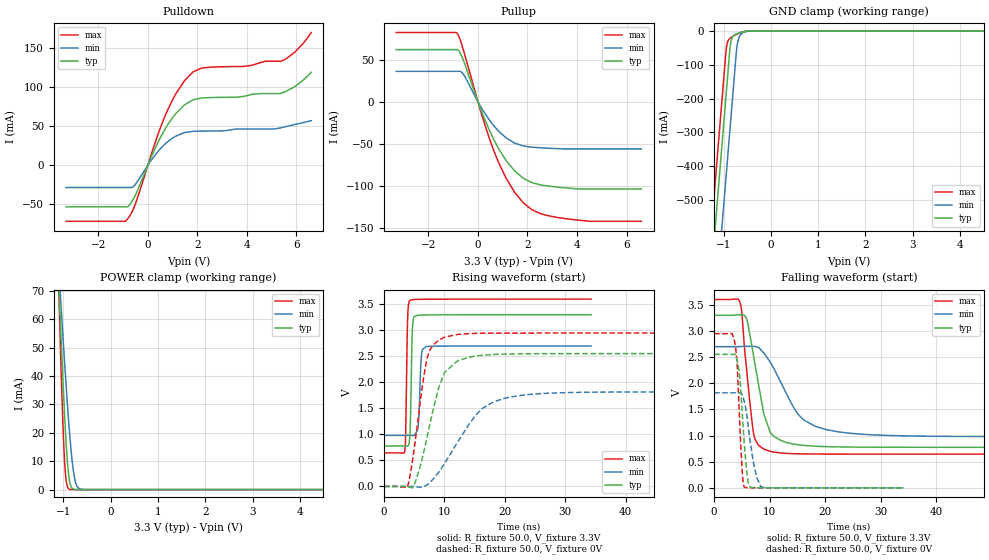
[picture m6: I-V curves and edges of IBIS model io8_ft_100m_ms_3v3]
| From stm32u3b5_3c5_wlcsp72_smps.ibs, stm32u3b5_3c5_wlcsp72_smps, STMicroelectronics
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[Model]   io8_ft_100m_ms_3v3
Model_type I/O
Polarity   Non-Inverting
Enable   Active-Low
| CAP_THRESHOLD on pad IOFT is "UDTCAPC" :
| Rising=30.0% of vddiom   Falling=70.0% of vddiom
| C_comp min and max val. don't necessarily correlate with the min and max pvt
| but are the smallest and greatest pad capacitance found.
| var   typ   min   max
C_comp   3.79549pF  3.74406pF  3.79817pF
|C_comp_pullup   2.32784pF  2.17308pF  2.40204pF
|C_comp_pulldown   1.46765pF  1.57099pF  1.39613pF
Vinl = 1.35V
Vinh = 1.8V
Vmeas = 1.65V   | Reference voltage for timing measurements
Cref  = 50.0pF   | Timing specification test load capacitance value
Rref  = 1.0MOhm   | Timing specification test load resistance value
Vref  = 1.815V   | Timing specification test load voltage
[Model Spec]
| TIME_THRESHOLD on pin ZIV11 is "CMOS" :
| Rising=50.0% of vdd   Falling=50.0% of vdd
Vinl 1.27950V 1.06950V 1.36550V
Vinh 1.78950V 1.51350V 1.89450V
| variable   typ   min   max
[Temperature Range] 25.0 130.0 -40.0
| variable   typ   min   max
[Voltage Range] 3.3V 2.7V 3.6V
| variable   typ   min   max
[POWER Clamp Reference] 3.3V 2.7V 3.6V
| variable   typ   min   max
[GND Clamp Reference] 0V 0V 0V
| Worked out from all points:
|   slope of the pulldown table from 0 to 0.495 V, typ, clamps not added: 14.3 ohm
|   slope of the pullup table from 0 to 0.495 V, typ, clamps not added: 13.8 ohm
|   GND clamp passes 1 mA (typ) near -0.50 V on its own axis
|   POWER clamp passes 1 mA (typ) near -0.83 V on its own axis
|   rising waveform, R_fixture 50.0, V_fixture 3.3V: 20-80 % time 257ps typ, 338ps min, 239ps max; typ from 0.776 V to 3.3 V
|   falling waveform, R_fixture 50.0, V_fixture 3.3V: 20-80 % time 2.72ns typ, 5.55ns min, 1.62ns max; typ from 3.3 V to 0.776 V
|   rising waveform, R_fixture 50.0, V_fixture 0V: 20-80 % time 3.27ns typ, 6.29ns min, 2.11ns max; typ from 0 V to 2.55 V
|   falling waveform, R_fixture 50.0, V_fixture 0V: 20-80 % time 1.01ns typ, 1.53ns min, 771ps max; typ from 2.55 V to 0 V
[POWER Clamp]
-3.3V     1.126A     769.5mA    1.647A
-1.1V     75.38mA    79.63mA    73.18mA
-1.09V    71.2mA     76.8mA     67.14mA
-1.08V    67.05mA    73.98mA    61.2mA
-1.06V    58.89mA    68.38mA    49.67mA
-1.01V    39.47mA    54.71mA    24.03mA
-970mV    25.49mA    44.18mA    9.257mA
-930mV    13.81mA    34.16mA    2.168mA
-870mV    3.251mA    20.56mA    140.6uA
-760mV    67.19uA    3.98mA     739.8nA
-630mV    518.7nA    149.1uA    1.803nA
6.6V      0A         0A         0A
[GND Clamp]
-3.3V     -4.191A    -4.432A    -4.059A
-1.25V    -706mA     -946.8mA   -573.6mA
-950mV    -196mA     -436.8mA   -63.63mA
-940mV    -179mA     -419.8mA   -50.26mA
-910mV    -128mA     -368.8mA   -31.05mA
-850mV    -37.37mA   -266.8mA   -20.53mA
-810mV    -18.79mA   -198.8mA   -16.88mA
-720mV    -8.735mA   -51.28mA   -10.12mA
-680mV    -6.635mA   -22.61mA   -7.598mA
-630mV    -4.51mA    -9.474mA   -4.925mA
-400mV    -114.4uA   -369.6uA   -46.93uA
6.6V      2.22nA     299.7nA    1.002nA
| variable   typ   min   max
[Pullup Reference] 3.3V 2.7V 3.6V
| variable   typ   min   max
[Pulldown Reference] 0V 0V 0V
[Pullup]
-3.3V     61.97mA    36.11mA    82.22mA
-840mV    61.97mA    36.11mA    81.38mA
-720mV    58.1mA     36.07mA    73.72mA
-570mV    48mA       31.88mA    59.76mA
170mV     -13.41mA   -8.675mA   -17.26mA
800mV     -53.86mA   -33.82mA   -69.73mA
1.14V     -69.93mA   -42.96mA   -90.97mA
1.48V     -82.17mA   -49.14mA   -107.6mA
2.17V     -96.08mA   -54mA      -128.2mA
2.85V     -100.3mA   -55.28mA   -135.6mA
3.88V     -103.2mA   -56.04mA   -140.2mA
6.6V      -103.8mA   -56.04mA   -142.1mA
[Pulldown]
-3.3V     -53.27mA   -28.52mA   -71.84mA
-840mV    -53.27mA   -28.52mA   -69.65mA
-500mV    -38.18mA   -24.47mA   -49.51mA
460mV     32.61mA    19.53mA    43.99mA
800mV     51.7mA     30.09mA    70.55mA
1.14V     66.56mA    37.47mA    92mA
1.48V     77.24mA    41.82mA    108.3mA
1.83V     83.91mA    43.43mA    119.6mA
2.17V     86.16mA    43.73mA    124.5mA
5.39V     92.36mA    48.12mA    133.3mA
5.93V     100.6mA    52.1mA     144.5mA
6.6V      119.1mA    57.05mA    170mA
[Ramp]
dV/dt_r 1.53142V/3.19498ns 1.09015V/6.22627ns 1.76896V/2.11107ns
dV/dt_f 1.51461V/2.56951ns 1.03188V/5.48087ns 1.77292V/1.61927ns
R_load = 50.0
| Removed startup time: 0s 0s 0s  .
| Removed end time: 34.25ns.
[Rising Waveform]
R_fixture   = 50.0
V_fixture   = 3.3V
V_fixture_min = 2.7V
V_fixture_max = 3.6V
0s        775.7mV    980.2mV    645.1mV
3.45ns    775.7mV    980.2mV    693.9mV
3.9ns     773.7mV    980.2mV    3.174V
4.3ns     998.1mV    980.2mV    3.573V
4.65ns    2.858V     979.9mV    3.587V
5ns       3.263V     977.5mV    3.593V
5.7ns     3.29V      1.21V      3.595V
6.25ns    3.294V     2.568V     3.597V
7ns       3.296V     2.691V     3.597V
34.25ns   3.3V       2.7V       3.6V
| Removed startup time: 0s 0s 0s  .
| Removed end time: 99.25ns.
[Falling Waveform]
R_fixture   = 50.0
V_fixture   = 3.3V
V_fixture_min = 2.7V
V_fixture_max = 3.6V
0s        3.3V       2.7V       3.6V
4.65ns    3.308V     2.699V     3.55V
5ns       3.308V     2.705V     3.354V
5.95ns    3.2V       2.706V     2.169V
7.2ns     2.471V     2.705V     997.4mV
9ns       1.401V     2.577V     739.2mV
10.15ns   1.052V     2.399V     697.1mV
15.1ns    824.5mV    1.411V     651mV
22.3ns    783.2mV    1.072V     645.7mV
99.25ns   775.7mV    980.2mV    645.1mV
| Removed startup time: 0s 0s 0s  .
| Removed end time: 99.2ns.
[Rising Waveform]
R_fixture   = 50.0
V_fixture   = 0V
V_fixture_min = 0V
V_fixture_max = 0V
0s        11.22nV    82.64nV    22.9nV
3.85ns    -3.742mV   1.837uV    -19.12mV
5.05ns    45.91mV    -1.708mV   765.4mV
7.15ns    956.6mV    31.23mV    2.467V
9.1ns     1.912V     278.7mV    2.815V
10.15ns   2.208V     463.1mV    2.872V
12.4ns    2.424V     895.1mV    2.923V
16.2ns    2.52V      1.494V     2.944V
22.3ns    2.548V     1.745V     2.948V
99.2ns    2.552V     1.817V     2.948V
| Removed startup time: 0s 0s 0s  .
| Removed end time: 34.2ns.
[Falling Waveform]
R_fixture   = 50.0
V_fixture   = 0V
V_fixture_min = 0V
V_fixture_max = 0V
0s        2.552V     1.817V     2.948V
3.7ns     2.556V     1.817V     2.797V
4.15ns    2.437V     1.817V     2.365V
4.65ns    2.097V     1.818V     1.176V
5.15ns    1.312V     1.756V     203.1mV
5.45ns    844mV      1.652V     16.71mV
6.3ns     46.27mV    1.053V     2.35mV
7.15ns    3.513mV    454.2mV    1.454mV
8.4ns     1.644mV    27.21mV    973.5uV
34.2ns    6.043uV    55.79uV    790.4nV
